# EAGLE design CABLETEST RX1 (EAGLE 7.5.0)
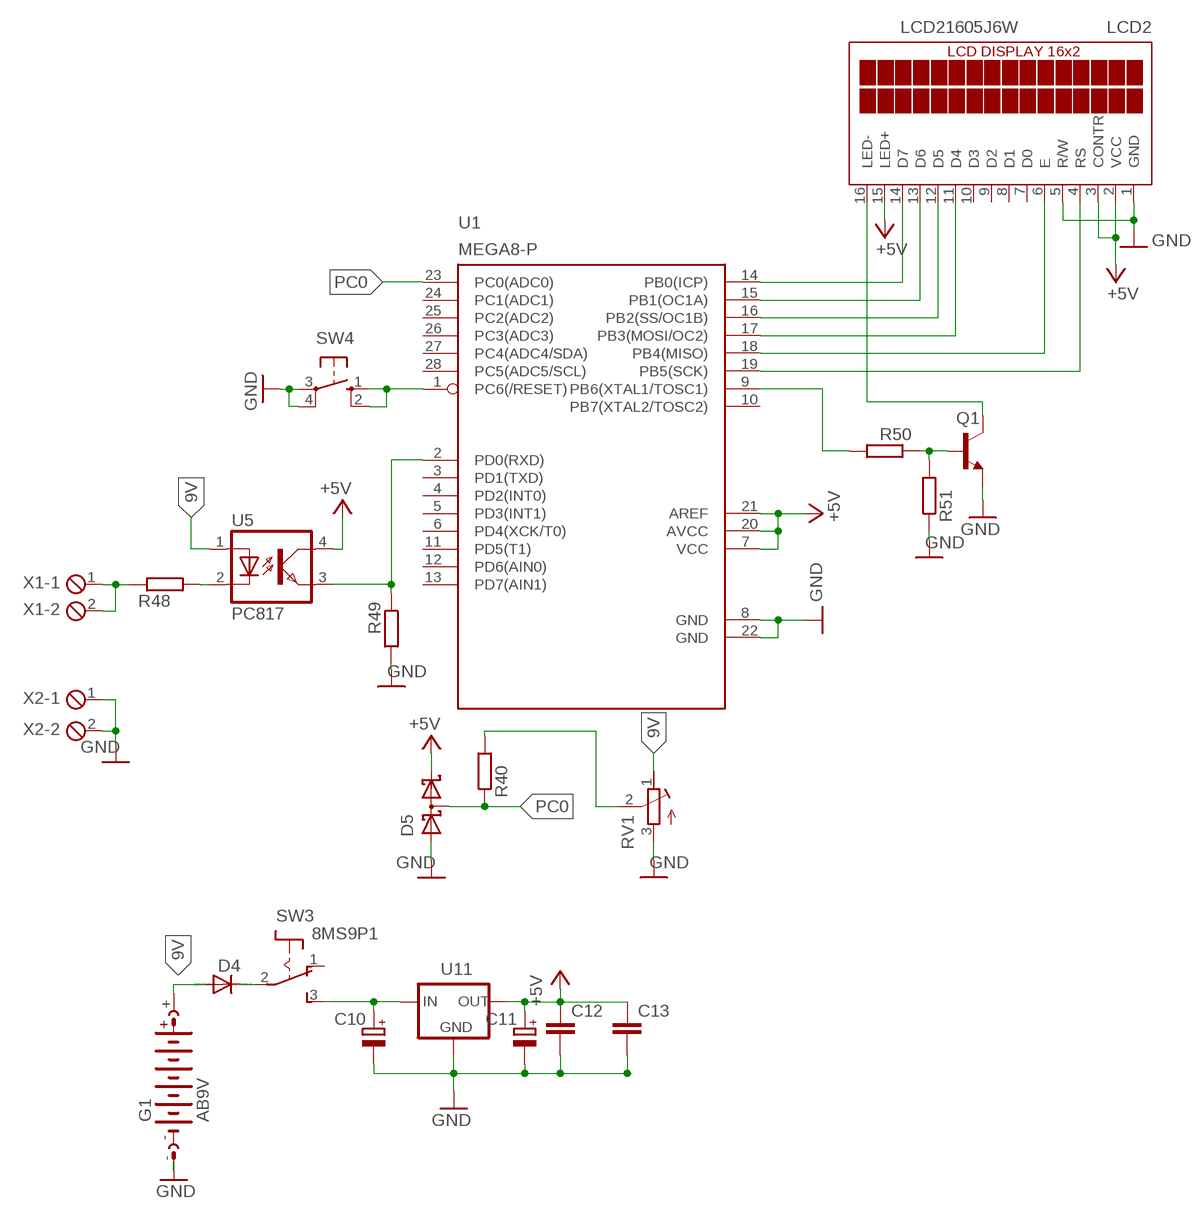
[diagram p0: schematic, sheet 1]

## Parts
C10  CPOL-EUE2-5  [E2-5]
C11  CPOL-EUE2-5  [E2-5]
C12  C-EUC1206  [C1206]
C13  C-EUC1206  [C1206]
D4  1N4004  [DO41-10]
D5  BAT54S  [SOT23]
G1  AB9V  [AB9V]
LCD2  LCD21605J6W  [LCD21605J6W]
Q1  BC337  [TO92]
R40  R-EU_M1206  [M1206]
R48  R-EU_M1206  [M1206]
R49  R-EU_M1206  [M1206]
R50  R-EU_M1206  [M1206]
R51  R-EU_M1206  [M1206]
RV1  R-TRIMM-3386-F  [R-TRIMM-3386F]
SW3  8MS9P1  [8MS9]
SW4  10-XX  [B3F-10XX]
U1  MEGA8-P  [DIL28-3]
U5  PC817  [DIL04]
U11  78XXL  [78XXL]
X1  MPT2  [2POL254]
X2  MPT2  [2POL254]

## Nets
9V: D4.A G1.+ RV1.1(A) U5.1(A)
+5V: C11.+ C12.1 C13.1 D5.2(C2) LCD2.2(VCC) LCD2.3(CONTR) LCD2.15(LED+) U1.7(VCC) U1.20(AVCC) U1.21(AREF) U5.4(COL) U11.OUT
GND: C10.- C11.- C12.2 C13.2 D5.1(A1) G1.- LCD2.1(GND) LCD2.5(R/W) Q1.1(E) R49.2 R51.1 RV1.3(E) SW4.3(P) SW4.4(P1) U1.8(GND) U1.22(GND) U11.GND X2.1 X2.2
N$1: LCD2.14(D7) U1.14(PB0(ICP))
N$2: LCD2.13(D6) U1.15(PB1(OC1A))
N$3: LCD2.12(D5) U1.16(PB2(SS/OC1B))
N$4: LCD2.11(D4) U1.17(PB3(MOSI/OC2))
N$5: LCD2.6(E) U1.18(PB4(MISO))
N$6: LCD2.4(RS) U1.19(PB5(SCK))
N$7: R49.1 U1.2(PD0(RXD)) U5.3(EMIT)
N$8: R48.2 U5.2(C)
N$10: D4.C SW3.2(P)
N$11: R40.2 RV1.2(S)
N$12: R48.1 X1.1 X1.2
N$13: C10.+ SW3.3(S) U11.IN
N$37: LCD2.16(LED-) Q1.3(C)
N$38: Q1.2(B) R50.1 R51.2
N$39: R50.2 U1.9(PB6(XTAL1/TOSC1))
N$40: SW4.1(S) SW4.2(S1) U1.1(PC6(/RESET))
PC0: D5.3(C1A2) R40.1 U1.23(PC0(ADC0))
Unconnected: LCD2.7(D0) LCD2.8(D1) LCD2.9(D2) LCD2.10(D3) SW3.1(O) U1.3(PD1(TXD)) U1.4(PD2(INT0)) U1.5(PD3(INT1)) U1.6(PD4(XCK/T0)) U1.10(PB7(XTAL2/TOSC2)) U1.11(PD5(T1)) U1.12(PD6(AIN0)) U1.13(PD7(AIN1)) U1.24(PC1(ADC1)) U1.25(PC2(ADC2)) U1.26(PC3(ADC3)) U1.27(PC4(ADC4/SDA)) U1.28(PC5(ADC5/SCL))

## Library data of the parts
C10 C11 = rcl:CPOL-EU: POLARIZED CAPACITOR, European symbol
C12 C13 = rcl:C-EU: CAPACITOR, European symbol
D4 = diode:1N4004: DIODE
D5 = diode:BAT54S: Schottky Diodes Pin connection corrected 2011-05-04 Source: Fairchild .. BAT54.pdf
G1 = battery:AB9V: 9-V BATTERY CLIP
LCD2 = display-lcd:LCD21605J6W
Q1 = transistor:BC337: NPN TRANSISTOR
R40 R48-R51 = resistor:R-EU_: RESISTOR, European symbol
RV1 = rcl:R-TRIMM-3386-F
SW3 = switch:8MS9P1
SW4 = switch-omron:10-XX: OMRON SWITCH; MPN: B3F-1000; OC_FARNELL: 176432; OC_NEWARK: 36M3542
U1 = atmel:MEGA8-P: MICROCONTROLLER 8 Kbytes FLASH, 1 kbytes SRAM, 512 bytes EEPROM, USART, 4-channel 10 bit ADC, 2-channel 8 bit ADC Pin compatible with Atmega48, ATMega88, ATMega168 Source: avr.lbr; OC_FARNELL: unknown; OC_NEWARK: unknown
U5 = optocoupler:PC817: SHARP OPTO COUPLER; MPN: PC817X4J000F; OC_FARNELL: 9707727; OC_NEWARK: 97K7059
U11 = v-reg:78XXL: VOLTAGE REGULATOR
X1 X2 = con-phoenix-254:MPT2: PHOENIX CONNECTOR; OC_FARNELL: unknown; OC_NEWARK: unknown

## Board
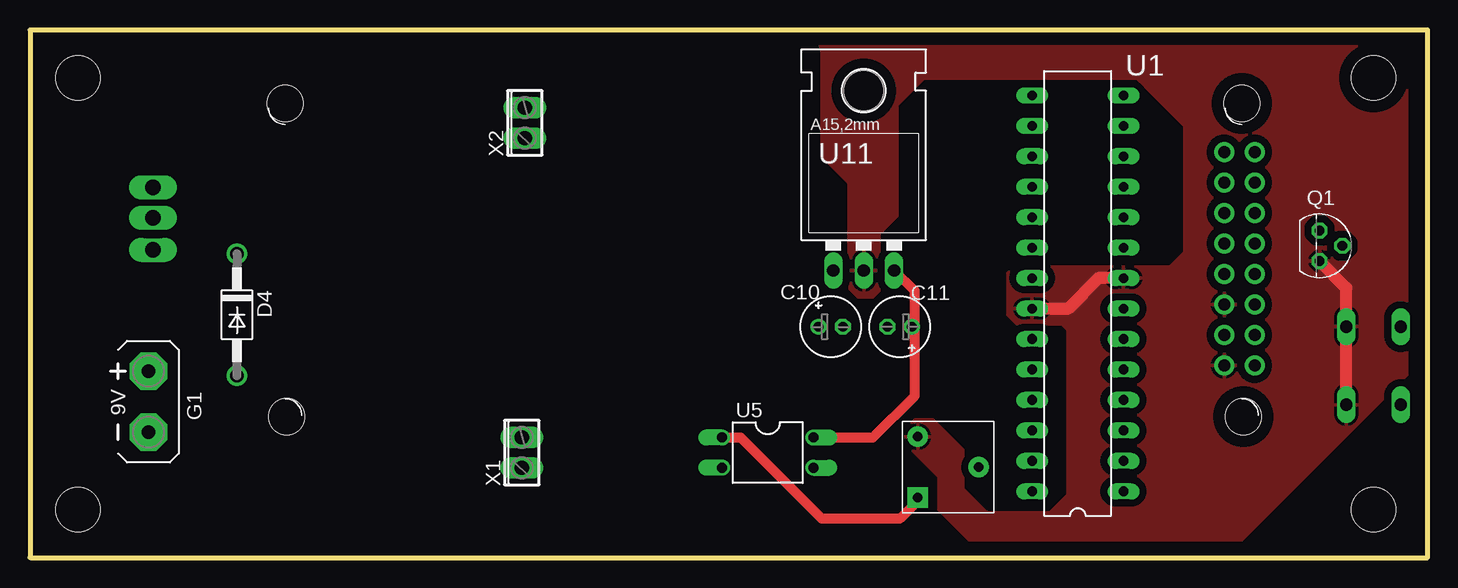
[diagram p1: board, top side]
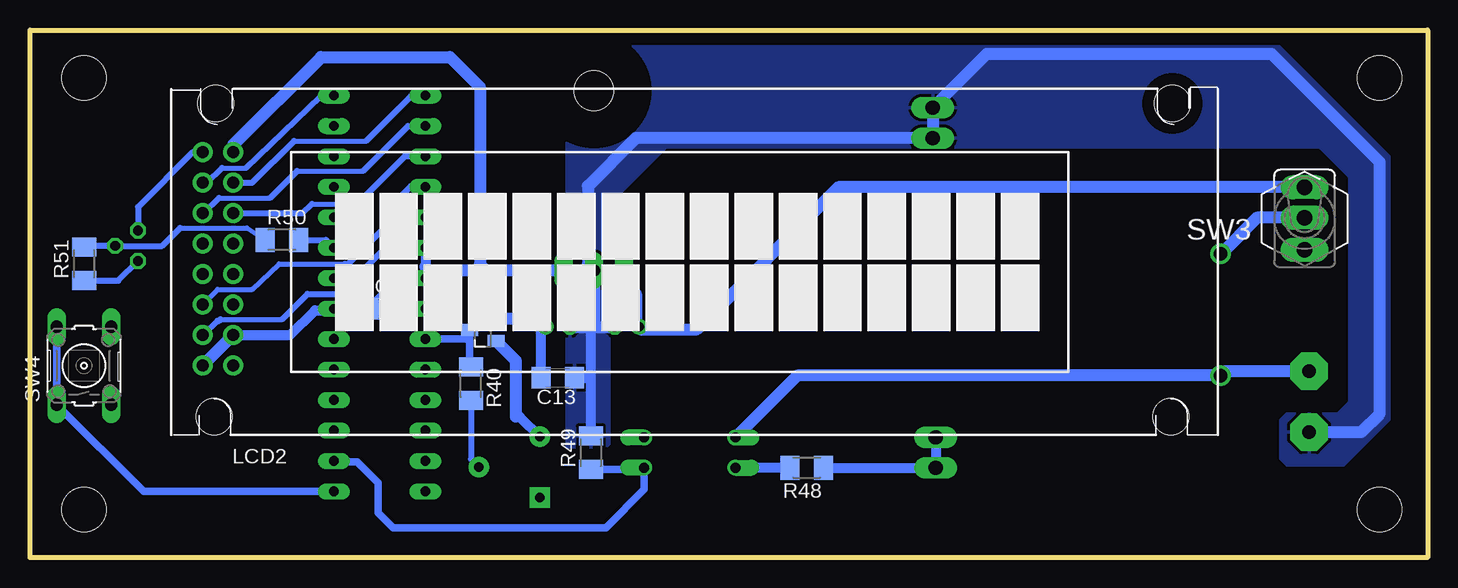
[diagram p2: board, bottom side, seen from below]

Size 116.5 x 44 mm. Coordinates in mm from the lower left corner, seen from the top.
Outline: 0,0 116.5,0 116.5,44 0,44 0,0
Copper layers (1*16): Top 0.035mm / dielectric 1.5mm / Bottom 0.035mm
Design rules "default": minimum track width 10mil, minimum drill 24mil, track to track 8mil, track to pad 8mil, pad to pad 8mil, via to via 8mil, smd to smd 8mil, copper to edge 40mil, drill to drill 8mil, minimum pad ring 10mil, minimum via ring 8mil, stop-mask expansion 4mil, vias tented up to drill 0mil, thermal gap 10mil
Holes 3.7 mm at 4,40 4,4 112,40 112,4

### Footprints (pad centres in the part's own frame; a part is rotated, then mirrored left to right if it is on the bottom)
E2-5 = drill 0.813 pad 1.27: + -1.016,0 | drill 0.813 pad 1.27 octagon: - 1.016,0
C1206 = smd 1.6 x 1.8: 1 -1.4,0; 2 1.4,0
DO41-10 = drill 1.118: A 5.08,0; C -5.08,0
SOT23 = smd 1 x 1.4: 1 -0.95,-1.1; 2 0.95,-1.1; 3 0,1.1
AB9V = drill 1.118 pad 3.15 octagon: + 0,2.54; - 0,-2.54
LCD21605J6W = drill 1 pad 1.676: 1 2.47,-17.72; 2 -0.07,-17.72; 3 2.47,-15.18; 4 -0.07,-15.18; 5 2.47,-12.64; 6 -0.07,-12.64; 7 2.47,-10.1; 8 -0.07,-10.1; 9 2.47,-7.56; 10 -0.07,-7.56; 11 2.47,-5.02; 12 -0.07,-5.02; 13 2.47,-2.48; 14 -0.07,-2.48; 15 2.47,0.06; 16 -0.07,0.06 | hole 3: 0.875,-22; 1,4.125; 80.75,4.125; 80.625,-22
TO92 = drill 0.813 octagon: 1 1.27,0; 2 0,1.905; 3 -1.27,0
M1206 = smd 1.6 x 2: 1 -1.4,0; 2 1.4,0
R-TRIMM-3386F = drill 0.8 pad 1.676 square: 1 0,0 | drill 0.8 pad 1.676: 2 5.08,2.54; 3 0,5.08
8MS9 = drill 1.295 pad 2 long: 1 -3,5.346 | drill 1.3 pad 2 long: 2 -3,2.654; 3 -3,0.114
B3F-10XX = drill 1.016 long: 1 -3.251,2.261; 2 3.251,2.261; 3 -3.251,-2.261; 4 3.251,-2.261
DIL28-3 = drill 0.813 long: 1 -16.51,-3.81; 2 -13.97,-3.81; 3 -11.43,-3.81; 4 -8.89,-3.81; 5 -6.35,-3.81; 6 -3.81,-3.81; 7 -1.27,-3.81; 8 1.27,-3.81; 9 3.81,-3.81; 10 6.35,-3.81; 11 8.89,-3.81; 12 11.43,-3.81; 13 13.97,-3.81; 14 16.51,-3.81; 15 16.51,3.81; 16 13.97,3.81; 17 11.43,3.81; 18 8.89,3.81; 19 6.35,3.81; 20 3.81,3.81; 21 1.27,3.81; 22 -1.27,3.81; 23 -3.81,3.81; 24 -6.35,3.81; 25 -8.89,3.81; 26 -11.43,3.81; 27 -13.97,3.81; 28 -16.51,3.81
DIL04 = drill 0.813 offset: 1 -1.27,-3.81; 2 1.27,-3.81; 3 1.27,3.81; 4 -1.27,3.81
78XXL = drill 1.016 long: GND 0,-3.81; IN -2.54,-3.81; OUT 2.54,-3.81 | hole 3.302: 0,11.176
2POL254 = drill 1.2 long: 1 -1.27,0; 2 1.27,0

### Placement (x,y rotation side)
C10  66.75,19.25 0 top
C11  72.5,19.25 180 top
C12  86.5,20.75 0 bottom
C13  72.5,15 0 bottom
D4  17.25,20.25 270 top
D5  78.75,19 90 bottom
G1  9.88,13 0 top
LCD2  102.02,33.75 0 bottom
Q1  107.5,26 270 top
R40  79.75,14.5 270 bottom
R48  51.75,7.5 180 bottom
R49  69.75,8.75 90 bottom
R50  95.5,26.5 0 bottom
R51  112,24.5 90 bottom
RV1  74,5 0 top
SW3  13.25,31 180 bottom
SW4  112,16 90 bottom
U1  87.35,22.03 90 top
U5  61.5,8.75 270 top
U11  69.5,27.75 0 top
X1  41,8.75 90 top
X2  41.25,36.25 90 top

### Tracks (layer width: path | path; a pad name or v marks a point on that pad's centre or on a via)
9V
  Top 0.813: RV1.1 74,4.75 72.5,3.25 66,3.25 59.25,10 57.71,10 U5.1
  Bottom 1.016: G1.+ 16.88,15.54 D4.A 52.54,15.17 U5.1
+5V
  Top 0.813: U5.4 70.27,10.02 73.75,13.5 73.75,22.23 U11.OUT
  Bottom 0.813: LCD2.3 94.81,18.57 92.75,20.62 91.3,20.62 U1.7 88.24,20.76 88,21 85.75,23.25 83.59,23.25 U1.21 83.54,24.25 U1.20 | C13.1 73.9,18.87 C11.+
  Bottom 1.016: LCD2.3 LCD2.2 | U11.OUT 77.75,23.94 | 77.75,23.94 78.5,23.94 | 78.5,23.94 83.23,23.94 83.54,24.25 | LCD2.15 99.55,34.45 92.25,41.75 81.5,41.75 79,39.25 79,24.44 78.5,23.94 | 77.75,23.94 77.65,23.84 D5.2 74.22,19.95 C11.+ | C12.1 87.9,20.9 88,21
GND
  Top 1.016: U1.8 89.05,23.3 86.5,20.75 U1.22 | Q1.1 109.74,22.49 SW4.4 SW4.3
  Bottom 0.5: R51.1 109.13,23.1 Q1.1
  Bottom 0.61: U1.22 C12.2
  Bottom 0.813: R49.2 69.75,15 | 69.75,15 69.75,19 70,19.25 | C13.2 69.75,15 | 76,11.75 75.67,11.75 RV1.3
  Bottom 1.016: 69.5,19.25 U11.GND 70,24.44 70,31 66.02,34.98 X2.1 X2.2 36.77,42 13,42 4,33 4,12 5.54,10.46 G1.- | 69.5,19.25 C10.- | C11.- 70,19.25 69.5,19.25 | 76,11.75 76,16.4 D5.1
  pour Bottom (isolate 0.61): 11.75,7.75 7,7.75 3.25,11.5 3.25,33.5 13,43.25 67.25,43.25 71.75,38.75 71.75,9.25 68.5,9.25 68.25,9.5 68.25,29.5 63.5,34.25 9,34.25 6.5,31.75 6.5,13 7.5,12 11.75,12 12.25,11.5 12.25,8.25
  pour Top (isolate 0.61): 68.25,28 68.25,31.25 66,33.5 66,42.5 65.75,42.75 113.75,42.75 114.75,41.75 114.75,15.25 101,1.5 78.25,1.5 75.75,4 75.75,6.75 73,9.5 73,10.75 73.75,11.5 75.25,11.5 77.75,9 77.75,5.75 79.75,3.75 85,3.75 86.5,5.25 86.5,19 86,19.5 82.25,19.5 81.5,20.25 81.5,23.75 82,24.25 95,24.25 96.25,25.5 96.25,36 92.25,40 74.5,40 72.25,37.75 72.25,28.5 70.75,27 70.75,22.25 70.25,21.75 69,21.75 68.25,22.5
N$1
  Bottom 0.406: 100.5,32.5 98.5,32.5
  Bottom 0.51: LCD2.14 101.73,31.27 100.5,32.5 | 98.5,32.5 92.25,38.5 91.2,38.5 U1.14
N$2
  Bottom 0.406: 94.5,34.75 88.5,34.75
  Bottom 0.51: LCD2.13 97.98,31.27 94.5,34.75 | 88.5,34.75 84.75,38.5 83.58,38.5 U1.15
N$3
  Bottom 0.4: 100.75,30 96.5,30
  Bottom 0.406: 94.25,32.25 88.75,32.25
  Bottom 0.51: LCD2.12 102.02,28.73 100.75,30 | 96.5,30 94.25,32.25 | 88.75,32.25 85,36 U1.16
N$4
  Bottom 0.406: 93,29.5 89.25,29.5
  Bottom 0.51: LCD2.11 93.77,28.73 93,29.5 | 89.25,29.5 85.25,33.5 83.58,33.5 U1.17
N$5
  Bottom 0.406: 84.12,30.88 83.58,30.88 U1.18 | LCD2.6 102.09,21.16 100.88,22.38 98,22.38 95.75,24.5 90.25,24.5
  Bottom 0.5: 90.25,24.5 90,24.5 87,27.5 87,28.75 84.75,31 83.62,31 U1.18
N$6
  Bottom 0.406: 100.62,19.88 95.5,19.88
  Bottom 0.51: LCD2.4 102.06,18.57 100.88,19.75 100.75,19.75 100.62,19.88 | 95.5,19.88 93.38,22 89.5,22 88.62,22.88 88.62,24.12 84.38,28.38 U1.19
N$7
  Bottom 0.61: U1.2 91.1,8 89.25,8 87.5,6.25 87.5,3.75 86.25,2.5 68.5,2.5 65.31,5.69 U5.3 65.44,7.35 R49.1
N$8
  Bottom 0.813: R48.2 57.67,7.5 U5.2
N$10
  Bottom 1.016: SW3.2 14.23,28.35 D4.C
N$11
  Bottom 0.5: R40.2 79.75,8.21 RV1.2
N$12
  Bottom 0.813: R48.1 41.02,7.5 X1.1 X1.2
N$13
  Bottom 1.016: SW3.3 49.11,30.89 61,19 65.48,19 C10.+ 66,19.52 66,22 66.96,22.96 U11.IN
N$37
  Bottom 0.5: LCD2.16 102.94,33.81 107.5,29.25 Q1.3
N$38
  Bottom 0.406: 104,27.5 98.4,27.5 R50.1
  Bottom 0.5: 104,27.5 105.5,26 Q1.2 111.9,26 R51.2
N$39
  Bottom 0.5: 91.32,26 U1.9 91.82,26.5 R50.2
N$40
  Bottom 0.61: U1.1 107.03,5.52 SW4.1 SW4.2
PC0
  Bottom 0.61: D5.3 79.85,18 | 79.85,18 79.85,16 R40.1 | U1.23 80.07,18.22 79.85,18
